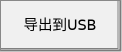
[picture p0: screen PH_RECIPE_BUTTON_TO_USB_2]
VISUALIZATION PH_RECIPE_BUTTON_TO_USB_2  // 122x52
VAR_IN_OUT
	RECIPE_CTRL_V2 : ST_RecipeCtrl_2;
END_VAR
    Button (0,0 120x50), "导出到USB", input disabled if: (RECIPE_CTRL_V2.sStatus.bBusy) <> 0, text list: 'TextList_Recipe', text index: 118
        p55702900: SEL(RECIPE_CTRL_V2.sCmd.bRecipeSaveToUSB, 16#000000, 16#00FF00)
        tap RECIPE_CTRL_V2.sCmd.bRecipeSaveToUSB
END_VISUALIZATION
